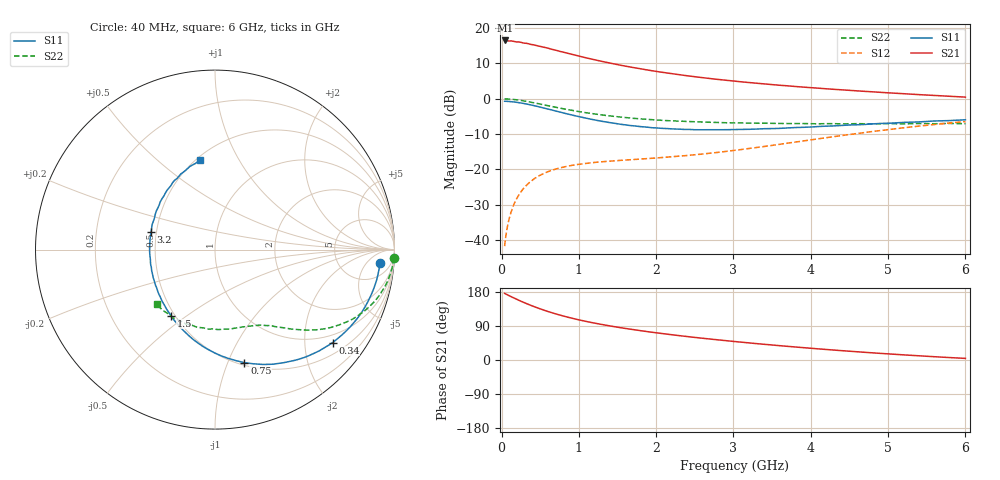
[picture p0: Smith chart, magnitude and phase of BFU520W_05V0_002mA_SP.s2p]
! Filename:  P:\Prog\Test\Noise\ATS_data\Testdata_Net\Run2\BFU520W_APM2013_06_A05_05p0V_002mA_SP_CM01_D.s2p
! Date/Time: Tue 26/Mar/2013 18:01:39
! BFU520W_APM2013_06_A05_05p0V_1to20mA_SP_CM01_Bias2_R.s2p
! MDIF S-parameter v. bias file
! BFU520W_APM2013_06_A05_05p0V_1to20mA_SP_CM01
! Date/time Thu Mar 21 14:22:37 2013
! VAR V_out= 4.9990
! VAR I_out= 2.0000
! VAR V_in= 0.8098
! VAR I_in= 0.0221
! Device data file deembeded for feedlines and parallel
! Original file: \Run2\BFU520W_APM2013_06_A05_05p0V_002mA_SP_CM01_R.s2p
! Feed-files: PR019V01_070313_Feed1.s2p, PR019V01_070313_Feed2.s2p
! Parallel-file: PR019V01_070313_Par.s2p
# MHz S MA R 50
!  Freq-MHz  S11-mag  S11-arg  S21-mag  S21-arg  S12-mag  S12-arg  S22-mag  S22-arg
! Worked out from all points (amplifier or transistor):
!   98 points, 40 MHz to 6 GHz, reference 50 ohm
!   highest |S21| = 16.5 dB at 50 MHz (marker M1)
!   |S21| within 3 dB of that: start of sweep to 740 MHz
!   unconditionally stable (mu >= 1): 2.369 GHz to 3.509 GHz
!   at 300 MHz: K = 0.18, MSG = 20.4 dB, |S12| = -25.0 dB
!   at 1.6 GHz: K = 0.79, MSG = 13.3 dB, |S12| = -17.4 dB
!   at 6 GHz: K = 0.82, MSG = 3.5 dB, |S12| = -6.5 dB
!   S11 on the Smith chart (normalised r, x): 40 MHz: 12, -12; 340 MHz: 0.78, -2.68; 750 MHz: 0.53, -1.15; 1.5 GHz: 0.48, -0.44; 3.2 GHz: 0.47, +0.11; 6 GHz: 0.52, +0.70
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40  0.9219 -4.7  6.682 175.9  0.00818 86.5  0.9969 -2.7
50  0.9213 -5.9  6.693 174.7  0.01015 86.1  0.9951 -3.4
90  0.9165 -10.5  6.574 170.5  0.01824 83.4  0.9912 -6.1
120  0.9102 -14.1  6.601 167.6  0.02411 81.3  0.9858 -8.0
220  0.8821 -25.4  6.374 158.1  0.04265 74.8  0.957 -14.3
340  0.8354 -38.3  6.043 147.5  0.06204 67.7  0.9106 -21.0
420  0.799 -46.3  5.784 141.0  0.07318 63.7  0.8765 -24.9
550  0.7376 -58.6  5.362 131.4  0.08785 58.0  0.8186 -30.4
600  0.7154 -63.2  5.211 128.0  0.09273 56.1  0.7976 -32.2
750  0.6509 -75.4  4.704 118.9  0.1045 51.5  0.7392 -36.9
900  0.5926 -86.7  4.284 110.8  0.1135 48.3  0.6897 -40.6
1050  0.5443 -97.0  3.901 103.8  0.1198 46.0  0.6449 -43.8
1250  0.4906 -109.5  3.474 95.5  0.1269 44.0  0.6004 -47.1
1500  0.4424 -123.8  3.046 86.6  0.1333 43.1  0.5568 -50.9
1800  0.403 -139.2  2.656 77.3  0.1401 43.9  0.5186 -54.7
2050  0.3827 -151.0  2.395 70.5  0.1464 45.4  0.4972 -57.8
2500  0.3645 -170.5  2.053 59.6  0.1611 48.8  0.4726 -64.0
3100  0.368 167.6  1.738 47.1  0.1911 53.8  0.4547 -73.3
3200  0.3693 164.3  1.698 45.2  0.1976 54.4  0.4519 -74.9
4100  0.4046 138.9  1.412 29.4  0.2715 56.3  0.4423 -92.1
5200  0.4626 114.3  1.18 13.6  0.3878 50.2  0.4409 -116.5
6000  0.5043 99.5  1.055 4.2  0.4756 42.4  0.4441 -136.5
